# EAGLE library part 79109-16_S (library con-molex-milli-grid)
RECEPTACAL
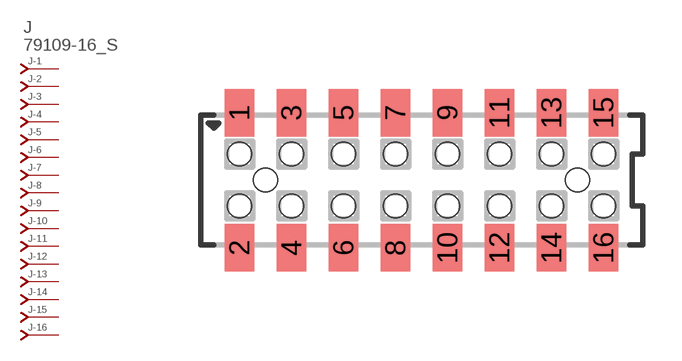
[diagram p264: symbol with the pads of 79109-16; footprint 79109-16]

Designator prefix J; gates -1=J-NV -2=J-N -3=J-N -4=J-N -5=J-N -6=J-N -7=J-N -8=J-N -9=J-N -10=J-N -11=J-N -12=J-N -13=J-N -14=J-N -15=J-N -16=J-N

## 79109-16_S  [79109-16]
1  -1:J  pas
2  -2:J  pas
3  -3:J  pas
4  -4:J  pas
5  -5:J  pas
6  -6:J  pas
7  -7:J  pas
8  -8:J  pas
9  -9:J  pas
10  -10:J  pas
11  -11:J  pas
12  -12:J  pas
13  -13:J  pas
14  -14:J  pas
15  -15:J  pas
16  -16:J  pas

## Footprint 79109-16 (pad centres in mm)
RECEPTACAL SMD Dual Row, Vertical, Pass-Thru
smd 1.12 x 1.83: 1 -7,2.6; 2 -7,-2.6; 3 -5,2.6; 4 -5,-2.6; 5 -3,2.6; 6 -3,-2.6; 7 -1,2.6; 8 -1,-2.6; 9 1,2.6; 10 1,-2.6; 11 3,2.6; 12 3,-2.6; 13 5,2.6; 14 5,-2.6; 15 7,2.6; 16 7,-2.6
hole 0.914 at -6,0
hole 0.914 at -7,1
hole 0.914 at -7,-1
hole 0.914 at -5,-1
hole 0.914 at -5,1
hole 0.914 at -3,-1
hole 0.914 at -3,1
hole 0.914 at 6,0
hole 0.914 at -1,1
hole 0.914 at -1,-1
hole 0.914 at 1,1
hole 0.914 at 1,-1
hole 0.914 at 3,1
hole 0.914 at 3,-1
hole 0.914 at 5,1
hole 0.914 at 5,-1
hole 0.914 at 7,-1
hole 0.914 at 7,1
